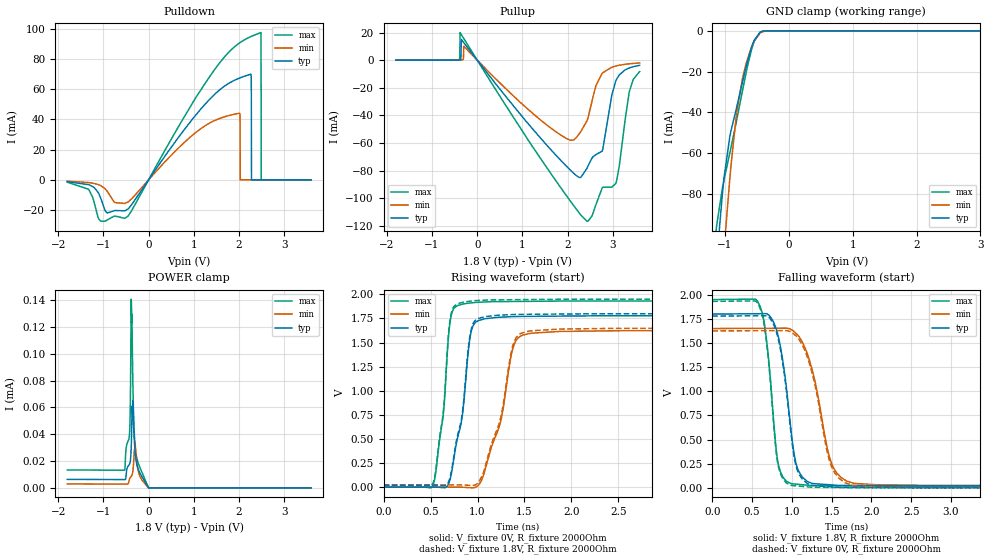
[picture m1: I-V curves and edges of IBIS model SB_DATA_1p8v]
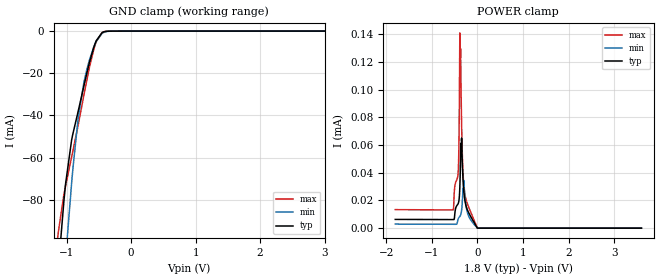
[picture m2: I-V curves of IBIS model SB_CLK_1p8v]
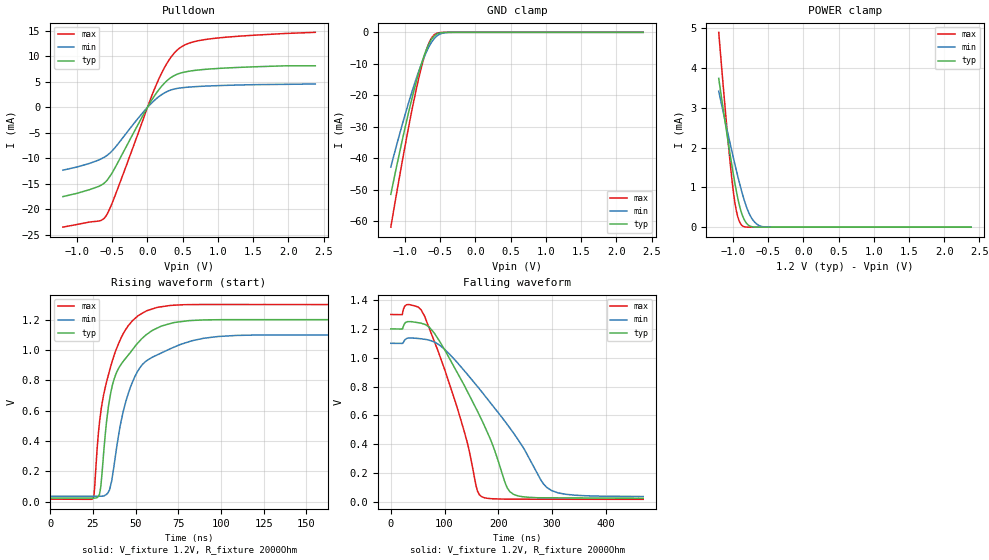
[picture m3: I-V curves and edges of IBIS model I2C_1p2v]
|Texas Instruments Incorporated
|Ultra Low Power Stereo Audio Codec with miniDSP, DirectPath Headphone,
| and Stereo Class-D Speaker Amplifier
|part#   Digital Voltage Range   Package-type   #pin
|TLV320AIC3263   1.1V to 3.6V   WCSP   81
[IBIS Ver]   4.1
[File name]   tlv320aic3263.ibs
[File Rev]   1.0
[Date]   03/05/2013
[Source]   Texas Instruments Incorporated.
   Analog-eLab, HPA
   12500 TI Blvd
   Dallas, TX -75243
   For Support e-mail: elab_ibis@list.ti.com
[Notes]   Revision History:
   1.0: 03/05/2011
- Initial version of the model
- Initial Model generated from simulations.
- Model not matched to measurements
- ccomp values are based on PVT conditions although listed in numerical order.
- Model names with a trailing _1p2v contains the model for 1.2V operaton.
- Model names with a trailing _1p8v contains the model for 1.8V operaton.
- Model names with a trailing _2p5v contains the model for 2.5V operaton.
- Model names with a trailing _3p3v contains the model for 3.3V operaton.
- Warnings regarding pull down/pull up and combined Non-monotonicity of various models
  have been reviewd and considered minor and can be ignored.
[Disclaimer]
 This product is designed as an aid for customers of Texas Instruments.
 No warranties, either expressed or implied, with respect to this third
 party software (if any) or with respect to its fitness for any
 particular purpose is claimed by Texas Instruments or the author. The
 software (if any) is provided solely on an "as is" basis. The entire
 risk as to its quality and performance is with the customer
[Copyright] (C) Copyright 2013 Texas Instruments Incorporated.
   All rights reserved.
|   TLV320AIC3263
[Component]   tlv320aic3263
[Manufacturer] TI
[Package]   | 81 pin  package
| variable   typ   min   max
R_pkg   0.01   0.008   0.012
L_pkg   0.1nH   0.08nH   0.12nH
C_pkg   0.1pF   0.08pF   0.12pF
|-------------------------PIN------------------------------------------------
[Pin]   signal_name  model_name  R_pin  L_pin C_pin
A1   MICBIAS_VDD   POWER   NA   NA   NA
A2   RECVSS   GND   NA   NA   NA
A3   RECVDD_33   POWER   NA   NA   NA
A4   HPR   TERM   NA   NA   NA
A5   VNEG   TERM   NA   NA   NA
A6   CPFCM   TERM   NA   NA   NA
A7   CPVDD_18   POWER   NA   NA   NA
A8   AVSS4   GND   NA   NA   NA
A9   SPKP   TERM   NA   NA   NA
B1   MICDET   TERM   NA   NA   NA
B2   RECP   TERM   NA   NA   NA
B3   RECM   TERM   NA   NA   NA
B4   HVDD_18   POWER   NA   NA   NA
B5   HPL   TERM   NA   NA   NA
B6   CPVSS   GND   NA   NA   NA
B7   CPFCP   TERM   NA   NA   NA
B8   SVDD   POWER   NA   NA   NA
B9   SVSS   GND   NA   NA   NA
C1   IN4L   TERM   NA   NA   NA
C2   AVDD1_18   POWER   NA   NA   NA
C3   MICBIAS_EXT   TERM   NA   NA   NA
C4   MICBIAS   TERM   NA   NA   NA
C5   AVDD2_18   POWER   NA   NA   NA
C6   LOL   TERM   NA   NA   NA
C7   AVDD4_18   POWER   NA   NA   NA
C8   SPKM   TERM   NA   NA   NA
C9   SPK_V   TERM   NA   NA   NA
D1   VREF_AUDIO   TERM   NA   NA   NA
D2   VREF_SAR   TERM   NA   NA   NA
D3   IN1L_AUX1   TERM   NA   NA   NA
D4   IN1R_AUX2   TERM   NA   NA   NA
D5   IN4R   TERM   NA   NA   NA
D6   HPVSS_SENSE   TERM   NA   NA   NA
D7   LOR   TERM   NA   NA   NA
D8   VBAT   TERM   NA   NA   NA
D9   DVSS   GND   NA   NA   NA
E1   IN3R   TERM   NA   NA   NA
E2   IN3L   TERM   NA   NA   NA
E3   AVSS   GND   NA   NA   NA
E4   AVSS1   GND   NA   NA   NA
E5   AVSS3   GND   NA   NA   NA
E6   AVSS2   GND   NA   NA   NA
E7   IOVDD_SB   POWER   NA   NA   NA
E8   DOUT2   TERM   NA   NA   NA
E9   SB_DATA   SB_DATA   NA   NA   NA
F1   IN2L   TERM   NA   NA   NA
F2   IN2R   TERM   NA   NA   NA
F3   AVDD_18   POWER   NA   NA   NA
F4   DVSS   GND   NA   NA   NA
F5   I2C_ADDR_SCLK   IN   NA   NA   NA
F6   SPI_SELECT   IN_PD   NA   NA   NA
F7   GPIO3   INOUT   NA   NA   NA
F8   GPIO4   INOUT   NA   NA   NA
F9   SB_CLK   SB_CLK   NA   NA   NA
G1   MCLK1   IN   NA   NA   NA
G2   GPIO1   INOUT   NA   NA   NA
G3   GPIO2   INOUT   NA   NA   NA
G4   RESETB   IN   NA   NA   NA
G5   GPIO6   INOUT   NA   NA   NA
G6   GPO1   OUT   NA   NA   NA
G7   DOUT3   OUT_HOLD   NA   NA   NA
G8   IOVSS   TERM   NA   NA   NA
G9   BCLK2   INOUT   NA   NA   NA
H1   BCLK1   INOUT   NA   NA   NA
H2   DOUT1   OUT_HOLD   NA   NA   NA
H3   IOVDD1   POWER   NA   NA   NA
H4   SCL   I2C_IO   NA   NA   NA
H5   GPIO5   INOUT   NA   NA   NA
H6   IOVDD3   POWER   NA   NA   NA
H7   DIN3   IN   NA   NA   NA
H8   DIN2   IN   NA   NA   NA
H9   IOVDD2   POWER   NA   NA   NA
J1   DIN1   IN   NA   NA   NA
J2   WCLK1   INOUT   NA   NA   NA
J3   DVDD   POWER   NA   NA   NA
J4   IOVSS   GND   NA   NA   NA
J5   SDA   I2C_IO   NA   NA   NA
J6   BCLK3   INOUT   NA   NA   NA
J7   WCLK3   INOUT   NA   NA   NA
J8   WCLK2   INOUT   NA   NA   NA
J9   DVDD   POWER   NA   NA   NA
[Model Selector] SB_DATA
SB_DATA_1p8v   SB_DATA with 1.8V operation.
SB_DATA_1p2v   SB_DATA with 1.2V operation.
[Model Selector] SB_CLK
SB_CLK_1p8v   SB_DATA with 1.8V operation.
SB_CLK_1p2v   SB_DATA with 1.2V operation.
[Model Selector] I2C_IO
I2C_3p3v   I2C I/O with 3.3V operation.
I2C_2p5v   I2C I/O with 2.5V operation.
I2C_1p8v   I2C I/O with 1.8V operation.
I2C_1p2v   I2C I/O with 1.2V operation.
[Model Selector] IN
IN_3p3v   Input with 3.3V operation.
IN_2p5v   Input with 2.5V operation.
IN_1p8v   Input with 1.8V operation.
IN_1p2v   Input with 1.2V operation.
[Model Selector] IN_PD
IN_PD_3p3v  Input with 3.3V operation.
IN_PD_2p5v  Input with 2.5V operation.
IN_PD_1p8v  Input with 1.8V operation.
IN_PD_1p2v  Input with 1.2V operation.
[Model Selector] INOUT
INOUT_3p3v   I/O with 3.3V operation.
INOUT_2p5v   I/O with 2.5V operation.
INOUT_1p8v   I/O with 1.8V operation.
INOUT_1p2v   I/O with 1.2V operation.
[Model Selector] OUT
OUT_3p3v   Output with 3.3V operation.
OUT_2p5v   Output with 2.5V operation.
OUT_1p8v   Output with 1.8V operation.
OUT_1p2v   Output with 1.2V operation.
[Model Selector] OUT_HOLD
OUT_HOLD_3p3v   Output with 3.3V operation.
OUT_HOLD_2p5v   Output with 2.5V operation.
OUT_HOLD_1p8v   Output with 1.8V operation.
OUT_HOLD_1p2v   Output with 1.2V operation.
[Model Selector] TERM
TERM_3p3v   Termination with 3.3V operation.
TERM_2p5v   Termination with 2.5V operation.
TERM_1p8v   Termination with 1.8V operation.
TERM_1p2v   Termination with 1.2V operation.
|   TERM_1p2v
[Model]  TERM_1p2v
Model_type Terminator
C_comp   1fF   1fF   1fF
[Voltage Range]  1.2   1.1  1.3
[Temperature Range] 27   125   -40
|   TERM_1p8v
[Model]  TERM_1p8v
Model_type Terminator
C_comp   1fF   1fF   1fF
[Voltage Range]  1.8   1.65  1.95
[Temperature Range] 27   125   -40
|   TERM_2p5v
[Model]  TERM_2p5v
Model_type Terminator
C_comp   1fF   1fF   1fF
[Voltage Range]  2.5   2.25  2.75
[Temperature Range] 27   125   -40
|   TERM_3p3v
[Model]  TERM_3p3v
Model_type Terminator
C_comp   1fF   1fF   1fF
[Voltage Range]  3.3   2.7  3.6
[Temperature Range] 27   125   -40
| Models and submodels in the file (32): SB_DATA_1p8v (I/O), SB_DATA_1p2v (I/O), SB_CLK_1p8v (Input), SB_CLK_1p2v (Input), I2C_1p2v (I/O_open_drain), I2C_1p8v (I/O_open_drain), I2C_2p5v (I/O_open_drain), I2C_3p3v (I/O_open_drain), IN_1p2v (Input), IN_1p8v (Input), IN_2p5v (Input), IN_3p3v (Input), IN_PD_1p2v (Input), IN_PD_1p8v (Input), IN_PD_2p5v (Input), IN_PD_3p3v (Input), INOUT_1p2v (I/O), INOUT_1p8v (I/O), INOUT_2p5v (I/O), INOUT_3p3v (I/O), OUT_1p2v (Output), OUT_1p8v (Output), OUT_2p5v (Output), OUT_3p3v (Output), OUT_HOLD_1p2v (Output), OUT_HOLD_1p8v (Output), OUT_HOLD_2p5v (Output), OUT_HOLD_3p3v (Output), TERM_1p2v (Terminator), TERM_1p8v (Terminator), TERM_2p5v (Terminator), TERM_3p3v (Terminator)
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|   SB_DATA_1p8v
[Model]   SB_DATA_1p8v
Model_type   I/O
Polarity   Non-Inverting
Enable   Active-Low
Vinl = 0.54
Vinh = 1.26
Vmeas = 0.9
Vref = 1.8
Cref = 1pF
Rref = 2000
|   typ   min   max
C_comp   0.971pF   0.938pF   1.010pF
[Voltage Range]   1.8   1.65   1.95
[Temperature Range]   27   125   -40
[Pullup Reference]   1.8   1.65   1.95
[Pulldown Reference]   -0   -0   -0
[Power Clamp Reference]   1.8   1.65   1.95
[GND Clamp Reference]   -0   -0   -0
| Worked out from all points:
|   slope of the pulldown table from 0 to 0.27 V, typ, clamps not added: 22.9 ohm
|   slope of the pullup table from 0 to 0.27 V, typ, clamps not added: 23.8 ohm
|   GND clamp passes 1 mA (typ) near -0.46 V on its own axis
|   falling waveform, V_fixture 1.8V, R_fixture 2000Ohm: 20-80 % time 164ps typ, 243ps min, 125ps max; typ from 1.8 V to 0.02 V
|   rising waveform, V_fixture 0V, R_fixture 2000Ohm: 20-80 % time 146ps typ, 225ps min, 107ps max; typ from 0 V to 1.78 V
|   rising waveform, V_fixture 1.8V, R_fixture 2000Ohm: 20-80 % time 146ps typ, 225ps min, 107ps max; typ from 0.02 V to 1.8 V
|   falling waveform, V_fixture 0V, R_fixture 2000Ohm: 20-80 % time 163ps typ, 243ps min, 125ps max; typ from 1.78 V to 0 V
[Pulldown]
|   Voltage   I(typ)   I(min)   I(max)
-1.8V     -1.239mA   -902uA     -1.576mA
-450mV    -19.19mA   -14.57mA   -23.91mA
1.996V    67.21mA    44.06mA    90.32mA
2.023V    67.54mA    42.5mA     90.89mA
2.029V    67.6mA     -4.416uA   91mA
2.261V    69.94mA    8.944nA    94.86mA
2.272V    68.21mA    8.955nA    95mA
2.277V    168.5nA    8.961nA    95.07mA
2.482V    1.616nA    9.354nA    97.54mA
2.488V    1.622nA    9.367nA    97.47mA
2.493V    1.628nA    9.381nA    2.138uA
3.595V    4.438nA    15.26nA    745.7pA
[GND Clamp]
|   Voltage   I(typ)   I(min)   I(max)
-1.8V     -421.6mA   -468.1mA   -392.6mA
-1.13V    -112.7mA   -155.7mA   -95.33mA
-1.044V   -80.7mA    -118.8mA   -77.58mA
-1.017V   -72.29mA   -107.7mA   -73.32mA
-925.2mV  -51.87mA   -72.53mA   -59.86mA
-822.6mV  -38.07mA   -41.31mA   -44.61mA
-730.8mV  -25.67mA   -23.89mA   -29.91mA
-649.8mV  -15.2mA    -13.98mA   -17.61mA
-558mV    -5.766mA   -5.923mA   -6.41mA
-450mV    -701.9uA   -1.075mA   -633uA
-261mV    -18.65uA   -19.22uA   -25.39uA
3.595V    0A         0A         0A
[Pullup]
|   Voltage   I(typ)   I(min)   I(max)
-1.8V     1.584nA    9.234nA    154.7pA
-390.6mV  20.32uA    509.3nA    471.6uA
-379.8mV  54.13uA    822.1nA    19.97mA
-358.2mV  3.421mA    2.992uA    18.85mA
-352.8mV  15.02mA    4.286uA    18.57mA
-298.8mV  12.72mA    10.13mA    15.76mA
2.045V    -79.13mA   -57.85mA   -101.4mA
2.439V    -77.66mA   -43.11mA   -116.8mA
2.779V    -64.6mA    -9.133mA   -92.06mA
3.065V    -15.23mA   -4.265mA   -89.47mA
3.362V    -5.702mA   -2.681mA   -23.41mA
3.595V    -3.75mA    -2.066mA   -8.316mA
[POWER Clamp]
|   Voltage   I(typ)   I(min)   I(max)
-1.8V     6.322uA    2.922uA    13.36uA
-525.6mV  6.184uA    2.805uA    13.43uA
-417.6mV  18.06uA    6.903uA    43uA
-401.4mV  20.86uA    7.801uA    70.67uA
-385.2mV  29.75uA    8.475uA    140.7uA
-374.4mV  43.34uA    9.045uA    123uA
-369mV    52.8uA     9.435uA    129.4uA
-347.4mV  64.91uA    12.7uA     76.4uA
-298.8mV  27.03uA    34.39uA    31.23uA
-212.4mV  12.58uA    10.49uA    16.95uA
-1.8mV    88.84nA    71.93nA    128nA
3.595V    0A         0A         0A
[Ramp]
R_load = 2000
|   typ   min   max
dV/dt_r   1.0674/1.45878e-10   0.975475/2.25818e-10   1.159/1.06767e-10
dV/dt_f   1.06793/1.63363e-10   0.975638/2.42853e-10   1.15945/1.24825e-10
[Falling Waveform]
V_fixture = 1.8V
V_fixture_min = 1.65V
V_fixture_max = 1.95V
R_fixture = 2000Ohm
C_fixture = 0F
|   Time   V(typ)   V(min)   V(max)
0s        1.8V       1.65V      1.95V
594.2ps   1.804V     1.652V     1.891V
686.3ps   1.803V     1.653V     1.501V
823.2ps   1.589V     1.653V     274.3mV
993.8ps   564.7mV    1.639V     43.5mV
1.07ns    204.9mV    1.586V     37.1mV
1.196ns   65.24mV    1.385V     27.94mV
1.503ns   30.42mV    245.1mV    21.99mV
1.763ns   25.2mV     50.6mV     19.97mV
10ns      20.12mV    23.94mV    17.59mV
[Rising Waveform]
V_fixture = 0V
V_fixture_min = 0V
V_fixture_max = 0V
R_fixture = 2000Ohm
C_fixture = 0F
|   Time   V(typ)   V(min)   V(max)
0s        18.47nV    394.9nV    3.62nV
524ps     104.5uV    66.79uV    19.09mV
637ps     -5.535mV   81.11uV    773.9mV
707.8ps   80.84mV    90.08uV    1.718V
849.8ps   842.5mV    -1.574mV   1.9V
967ps     1.697V     -4.263mV   1.915V
1.232ns   1.762V     628.3mV    1.924V
1.391ns   1.769V     1.483V     1.926V
1.54ns    1.771V     1.591V     1.927V
10ns      1.779V     1.626V     1.932V
[Rising Waveform]
V_fixture = 1.8V
V_fixture_min = 1.65V
V_fixture_max = 1.95V
R_fixture = 2000Ohm
C_fixture = 0F
|   Time   V(typ)   V(min)   V(max)
0s        20.11mV    23.9mV     17.58mV
524ps     20.21mV    23.96mV    37.12mV
637ps     14.78mV    23.97mV    796mV
707.8ps   103mV      23.98mV    1.739V
849.8ps   870.6mV    22.42mV    1.919V
967ps     1.719V     20.31mV    1.934V
1.232ns   1.784V     662.2mV    1.943V
1.391ns   1.79V      1.514V     1.944V
1.54ns    1.793V     1.616V     1.945V
10ns      1.8V       1.65V      1.95V
[Falling Waveform]
|Gnd
V_fixture = 0V
V_fixture_min = 0V
V_fixture_max = 0V
R_fixture = 2000Ohm
C_fixture = 0F
|   Time   V(typ)   V(min)   V(max)
0s        1.779V     1.626V     1.932V
594.2ps   1.782V     1.628V     1.872V
686.3ps   1.781V     1.628V     1.477V
823.2ps   1.563V     1.629V     251.3mV
993.8ps   532mV      1.615V     25.65mV
1.129ns   92.82mV    1.485V     15.07mV
1.275ns   23.23mV    1.122V     6.102mV
1.503ns   10.16mV    211.8mV    4.346mV
1.763ns   5.019mV    25.84mV    2.341mV
10ns      12.68uV    25.78uV    5.568uV
|   SB_CLK_1p8v
[Model]   SB_CLK_1p8v
Model_type   Input
Vinl = 0.54
Vinh = 1.26
|   typ   min   max
C_comp   0.971pF   0.938pF   1.010pF
[Voltage Range]   1.8   1.65   1.95
[Temperature Range]   27   125   -40
[Power Clamp Reference]   1.8   1.65   1.95
[GND Clamp Reference]   -0   -0   -0
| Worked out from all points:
|   GND clamp passes 1 mA (typ) near -0.46 V on its own axis
[GND Clamp]
|   Voltage   I(typ)   I(min)   I(max)
-1.8V     -421.6mA   -468.1mA   -392.6mA
-1.13V    -112.7mA   -155.7mA   -95.33mA
-1.044V   -80.7mA    -118.8mA   -77.58mA
-1.017V   -72.29mA   -107.7mA   -73.32mA
-925.2mV  -51.87mA   -72.53mA   -59.86mA
-822.6mV  -38.07mA   -41.31mA   -44.61mA
-730.8mV  -25.67mA   -23.89mA   -29.91mA
-649.8mV  -15.2mA    -13.98mA   -17.61mA
-558mV    -5.766mA   -5.923mA   -6.41mA
-450mV    -701.9uA   -1.075mA   -633uA
-261mV    -18.65uA   -19.22uA   -25.39uA
3.595V    0A         0A         0A
[POWER Clamp]
|   Voltage   I(typ)   I(min)   I(max)
-1.8V     6.322uA    2.922uA    13.36uA
-525.6mV  6.184uA    2.805uA    13.43uA
-417.6mV  18.06uA    6.903uA    43uA
-401.4mV  20.86uA    7.801uA    70.67uA
-385.2mV  29.75uA    8.475uA    140.9uA
-374.4mV  43.34uA    9.045uA    123uA
-369mV    52.8uA     9.435uA    129.4uA
-347.4mV  64.91uA    12.7uA     76.4uA
-298.8mV  27.03uA    34.39uA    31.23uA
-212.4mV  12.58uA    10.49uA    16.95uA
-1.8mV    88.84nA    71.93nA    128nA
3.595V    0A         0A         0A
[Model]   I2C_1p2v
Model_type   I/O_open_drain
Polarity   Non-Inverting
Enable   Active-High
Vinl = 0.12
Vinh = 1.08
Vmeas = 0.6
Vref = 0
Cref = 5pF
Rref = 2000
|   typ   min   max
C_comp   1.274pF   1.219pF   1.333pF
[Voltage Range]   1.2   1.1   1.3
[Temperature Range]   27   125   -40
[Pullup Reference]   1.2   1.1   1.3
[Pulldown Reference]   -0   -0   -0
[Power Clamp Reference]   1.2   1.1   1.3
[GND Clamp Reference]   -0   -0   -0
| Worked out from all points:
|   slope of the pulldown table from 0 to 0.18 V, typ, clamps not added: 47.5 ohm
|   GND clamp passes 1 mA (typ) near -0.58 V on its own axis
|   POWER clamp passes 1 mA (typ) near -0.96 V on its own axis
|   falling waveform, V_fixture 1.2V, R_fixture 2000Ohm: 20-80 % time 88.3ns typ, 123ns min, 62.1ns max; typ from 1.2 V to 0.024 V
|   rising waveform, V_fixture 1.2V, R_fixture 2000Ohm: 20-80 % time 14.7ns typ, 15.2ns min, 13.1ns max; typ from 0.024 V to 1.2 V
[Pulldown]
|   Voltage   I(typ)   I(min)   I(max)
-1.2V     -17.52mA   -12.33mA   -23.52mA
-660mV    -15.3mA    -10.14mA   -22.22mA
-588mV    -14.55mA   -9.571mA   -21.32mA
-534mV    -13.56mA   -8.98mA    -19.87mA
-444mV    -11.44mA   -7.63mA    -16.76mA
-84mV     -2.1mA     -1.335mA   -3.236mA
132mV     2.914mA    1.776mA    4.67mA
294mV     5.441mA    3.206mA    9.049mA
456mV     6.677mA    3.793mA    11.64mA
636mV     7.195mA    4.032mA    12.81mA
924mV     7.575mA    4.234mA    13.51mA
2.382V    8.16mA     4.595mA    14.74mA
[GND Clamp]
|   Voltage   I(typ)   I(min)   I(max)
-1.2V     -51.53mA   -42.82mA   -61.95mA
-1.11V    -41.81mA   -35.22mA   -50.18mA
-966mV    -27.21mA   -23.77mA   -32.33mA
-894mV    -20.51mA   -18.48mA   -24.05mA
-822mV    -14.35mA   -13.57mA   -16.43mA
-750mV    -8.941mA   -9.16mA    -9.735mA
-696mV    -5.556mA   -6.287mA   -5.617mA
-642mV    -2.944mA   -3.902mA   -2.598mA
-588mV    -1.249mA   -2.113mA   -881.8uA
-498mV    -172.7uA   -521.4uA   -72.82uA
-372mV    -4.652uA   -38.41uA   -629.2nA
2.382V    0A         0A         0A
[POWER Clamp]
|   Voltage   I(typ)   I(min)   I(max)
-1.2V     3.742mA    3.419mA    4.901mA
-1.074V   2.231mA    2.387mA    2.298mA
-1.002V   1.428mA    1.82mA     1.03mA
-966mV    1.06mA     1.547mA    562.3uA
-930mV    731.2uA    1.283mA    261.4uA
-894mV    461.7uA    1.032mA    95.6uA
-858mV    267uA      798.5uA    24.83uA
-804mV    94.07uA    498uA      2.256uA
-732mV    11.82uA    224.2uA    69.47nA
-660mV    942.6nA    77.54uA    0A
-570mV    25.2nA     10.87uA    0A
2.382V    0A         0A         0A
[Ramp]
R_load = 2000
|   typ   min   max
dV/dt_r   0.705406/1.46932e-008  0.638454/1.52438e-008  0.769932/1.30398e-008
dV/dt_f   0.705409/8.81291e-008   0.63829/1.23398e-007  0.769933/6.21317e-008
[Falling Waveform]
V_fixture = 1.2V
V_fixture_min = 1.1V
V_fixture_max = 1.3V
R_fixture = 2000Ohm
C_fixture = 0F
|   Time   V(typ)   V(min)   V(max)
0s        1.2V       1.1V       1.3V
32.69ns   1.251V     1.136V     1.369V
62.72ns   1.232V     1.128V     1.29V
120.1ns   920.9mV    981.3mV    694.6mV
161.3ns   629.2mV    800.4mV    74.84mV
169.6ns   565.2mV    761.9mV    34.22mV
216.7ns   96.76mV    537mV      17.74mV
228.5ns   51.31mV    476.9mV    17.7mV
299.2ns   27.33mV    77.85mV    17.43mV
470ns     24.32mV    36.18mV    16.78mV
[Rising Waveform]
V_fixture = 1.2V
V_fixture_min = 1.1V
V_fixture_max = 1.3V
R_fixture = 2000Ohm
C_fixture = 0F
|   Time   V(typ)   V(min)   V(max)
0s        24.32mV    35.9mV     16.78mV
24.99ns   24.02mV    35.98mV    20.42mV
29.9ns    136.2mV    36mV       617.3mV
34.13ns   633.5mV    65.85mV    839.6mV
37.53ns   812.9mV    252.1mV    970.6mV
42.58ns   923.8mV    589mV      1.105V
48.06ns   1.001V     786.7mV    1.193V
62.72ns   1.146V     968.9mV    1.282V
109.1ns   1.201V     1.097V     1.301V
470ns     1.2V       1.1V       1.3V
